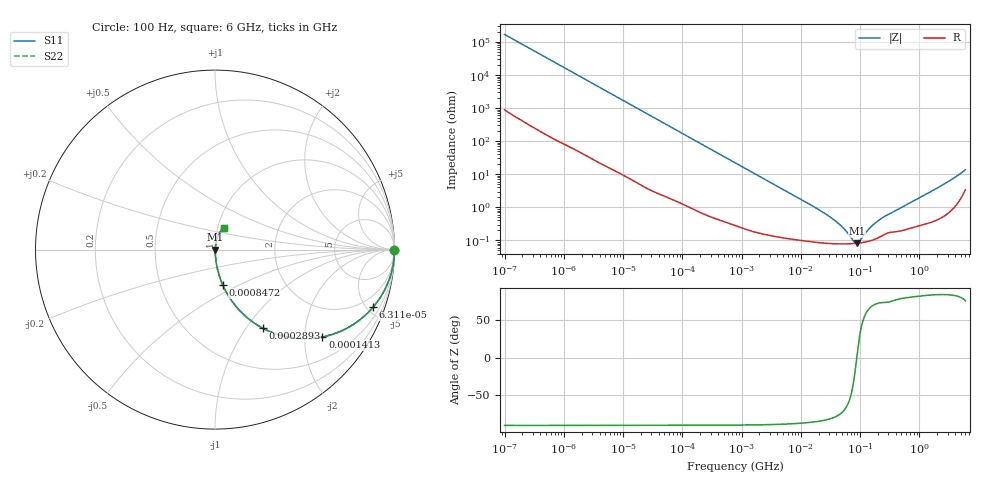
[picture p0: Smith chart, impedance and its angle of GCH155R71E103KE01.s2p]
!Murata Part Number: GCH155R71E103KE01
!These Parameters are Measured in Series Mode Connection
!Data Generated on Jun 19, 2026
!  o--ll--o
!Port1  Port2
!  o------o
!Operation Temp=25[degC], DC Bias Voltage=0[V]
!Freq. Start=100[Hz] Stop=6[GHz] 401[Steps]
# Hz S RI R 50
!Freq.(Hz) S11(Real) S11(Imag) S21(Real) S21(Imag) S12(Real) S12(Imag) S22(Real) S22(Imag)
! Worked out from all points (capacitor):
!   401 points, 100 Hz to 6 GHz, reference 50 ohm
!   read as one part in series: C = 9.43 nF near 109 Hz
!   lowest |Z| = 82.1 mohm at 89.18 MHz (marker M1)
!   series resonance near 87.89 MHz, so ESL is about 350 pH
!   S11 on the Smith chart (normalised r, x): 100 Hz: open; 63.12 kHz: 1.04, -5.45; 141.3 kHz: 1.02, -2.44; 289.3 kHz: 1.01, -1.20; 847.2 kHz: 1.01, -0.41; 6 GHz: 1.07, +0.27
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100  1 -0.000593  3.5e-06 0.000593  3.5e-06 0.000593  1 -0.000593
2008  0.9998 -0.0118  0.000199 0.0118  0.000199 0.0118  0.9998 -0.0118
12041  0.9947 -0.07  0.00531 0.07  0.00531 0.07  0.9947 -0.07
40335  0.9466 -0.222  0.0534 0.222  0.0534 0.222  0.9466 -0.222
63115  0.8797 -0.322  0.1203 0.322  0.1203 0.322  0.8797 -0.322
94437  0.7675 -0.4188  0.2325 0.4188  0.2325 0.4188  0.7675 -0.4188
141303  0.5982 -0.4865  0.4018 0.4865  0.4018 0.4865  0.5982 -0.4865
289253  0.2657 -0.4373  0.7343 0.4373  0.7343 0.4373  0.2657 -0.4373
452617  0.1307 -0.332  0.8693 0.332  0.8693 0.332  0.1307 -0.332
774597  0.0505 -0.2128  0.9495 0.2128  0.9495 0.2128  0.0505 -0.2128
847162  0.0429 -0.1963  0.9571 0.1963  0.9571 0.1963  0.0429 -0.1963
2713602  0.00559 -0.0641  0.9944 0.0641  0.9944 0.0641  0.00559 -0.0641
1.555665e7  0.00102 -0.0111  0.999 0.0111  0.999 0.0111  0.00102 -0.0111
3.983537e7  0.000797 -0.00358  0.9992 0.00358  0.9992 0.00358  0.000797 -0.00358
5.449875e7  0.000785 -0.00203  0.9992 0.00203  0.9992 0.00203  0.000785 -0.00203
7.797396e7  0.000802 -0.00049  0.9992 0.00049  0.9992 0.00049  0.000802 -0.00049
8.918374e7  0.000818 6.08e-05  0.9992 -6.08e-05  0.9992 -6.08e-05  0.000818 6.08e-05
9.753859e7  0.000834 0.000428  0.9992 -0.000428  0.9992 -0.000428  0.000834 0.000428
1.669249e8  0.00104 0.00278  0.999 -0.00278  0.999 -0.00278  0.00104 0.00278
3.124326e8  0.00176 0.00607  0.9982 -0.00607  0.9982 -0.00607  0.00176 0.00607
2.048624e9  0.0057 0.0385  0.9943 -0.0385  0.9943 -0.0385  0.0057 0.0385
6e9  0.0485 0.1222  0.9515 -0.1222  0.9515 -0.1222  0.0485 0.1222
